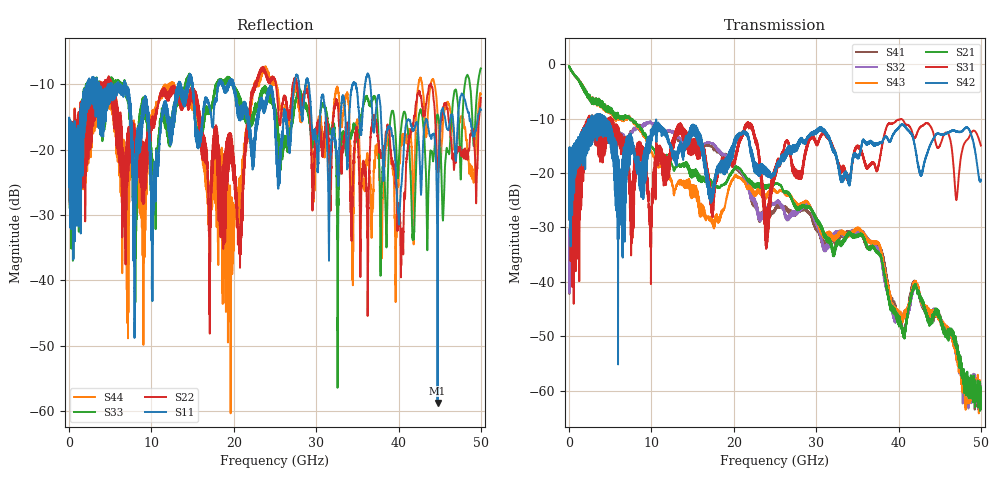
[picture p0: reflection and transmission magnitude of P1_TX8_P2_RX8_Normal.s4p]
!Keysight Technologies,N5225A,MY51441389,A.10.49.11
!Date: Monday, July 08, 2019 13:08:43
!Correction: S11(Full 4 Port(1,2,3,4))
!S12(Full 4 Port(1,2,3,4))
!S13(Full 4 Port(1,2,3,4))
!S14(Full 4 Port(1,2,3,4))
!S21(Full 4 Port(1,2,3,4))
!S22(Full 4 Port(1,2,3,4))
!S23(Full 4 Port(1,2,3,4))
!S24(Full 4 Port(1,2,3,4))
!S31(Full 4 Port(1,2,3,4))
!S32(Full 4 Port(1,2,3,4))
!S33(Full 4 Port(1,2,3,4))
!S34(Full 4 Port(1,2,3,4))
!S41(Full 4 Port(1,2,3,4))
!S42(Full 4 Port(1,2,3,4))
!S43(Full 4 Port(1,2,3,4))
!S44(Full 4 Port(1,2,3,4))
!S4P File: Measurements: <S11,S12,S13,S14>,
!<S21,S22,S23,S24>,
!<S31,S32,S33,S34>,
!<S41,S42,S43,S44>:
# Hz S  dB  R 50
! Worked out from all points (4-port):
!   5000 points, 10 MHz to 50 GHz, reference 50 ohm
!   strongest paths, dB at 10 MHz, 12.51 GHz, 25.01 GHz, 37.51 GHz, 50 GHz:
!     S42: -19.1, -16.6, -20.1, -14.7, -21.2
!     S31: -19.1, -16.0, -19.0, -19.0, -15.0
!     S21: -0.4, -18.5, -21.9, -34.7, -59.4
!     S43: -0.4, -21.8, -23.2, -33.0, -60.9
!     S32: -32.3, -12.3, -25.6, -34.2, -59.7
!     S41: -32.7, -12.2, -26.8, -33.7, -60.5
!   lowest |S11| = -58.8 dB at 44.74 GHz (marker M1), VSWR 1.00, Z = 50 + j0.114 ohm
!   |S11| at or under -10 dB: 6.882 GHz to 13.26 GHz (6.377 GHz wide, 63.3 % of centre); 20.01 GHz to 27.35 GHz (7.335 GHz wide, 31 % of centre); 36.58 GHz to end of sweep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
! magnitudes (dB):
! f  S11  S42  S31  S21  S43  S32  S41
! 10 MHz  -17.5  -19.1  -19.1  -0.4  -0.4  -32.3  -32.7
! 1.78 GHz  -12.1  -12.8  -13.9  -4.8  -4.7  -11.7  -11.6
! 9.82 GHz  -20.2  -14.9  -29.3  -14.7  -15.5  -10.5  -10.5
! 36.27 GHz  -8.3  -14.4  -18.9  -34.0  -32.7  -32.5  -33.9
! 41.79 GHz  -17.1  -13.6  -13.2  -41.1  -40.5  -41.8  -40.1
! 44.74 GHz  -58.8  -12.7  -15.4  -45.5  -46.4  -46.0  -46.0
! 50 GHz  -13.9  -21.2  -15.0  -59.4  -60.9  -59.7  -60.5
